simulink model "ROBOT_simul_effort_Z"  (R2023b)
settings: Solver=VariableStepAuto  StartTime=0.0  StopTime=5  RelTol=1e-3
undefined symbols (not defined in the file): deg, kg, m, manette1_Defaut_sldprt, manette2_Defaut_sldprt, mm, N, rad, s, STL, X, Y, Z
libraries: sm_lib x463, fl_lib x45, nesl_utility x27, simulink x2
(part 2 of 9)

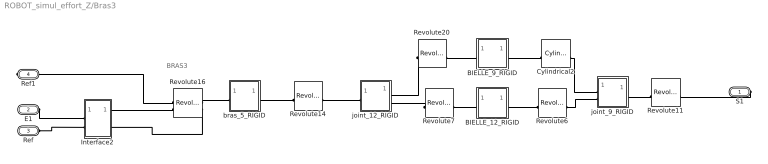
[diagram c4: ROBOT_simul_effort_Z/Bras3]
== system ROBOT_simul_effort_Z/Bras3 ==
  note: BRAS3
  BIELLE_12_RIGID : Subsystem
  BIELLE_9_RIGID : Subsystem
  Cylindrical2 : sm_lib/Joints/Cylindrical Joint  JointMode=Normal  SenseConstraintForce=off  SenseConstraintForceX=off  SenseConstraintForceY=off  SenseConstraintForceZ=off  SenseConstraintTorque=off  SenseConstraintTorqueX=off  SenseConstraintTorqueY=off  SenseConstraintTorqueZ=off  SenseTotalForce=off  SenseTotalForceX=off  SenseTotalForceY=off  SenseTotalForceZ=off  SenseTotalTorque=off  SenseTotalTorqueX=off  SenseTotalTorqueY=off  SenseTotalTorqueZ=off  CompositeWrenchDir=FollowerOnBase  CompositeWrenchFrame=BaseFrame  PzEquilibriumPosition=0  PzEquilibriumPositionUnits=m  PzSpringStiffness=0  PzSpringStiffnessUnits=N/m  PzDampingCoefficient=0  PzDampingCoefficientUnits=s*N/m  PzTorqueActuationMode=NoTorque  PzMotionActuationMode=ComputedMotion  PzSensePosition=off  PzSenseVelocity=off  PzSenseAcceleration=off  PzSenseTorqueForce=off  PzSenseLowerLimitTorqueForce=off  PzSenseUpperLimitTorqueForce=off  PzLowerLimitSpecify=off  PzLowerLimitBound=-1  PzLowerLimitBoundUnits=m  PzLowerLimitStiffness=1e6  PzLowerLimitStiffnessUnits=N/m  PzLowerLimitDamping=1e3  PzLowerLimitDampingUnits=N/(m/s)  PzLowerLimitTransitionRegionWidth=1e-4  PzLowerLimitTransitionRegionWidthUnits=m  PzUpperLimitSpecify=off  PzUpperLimitBound=1  PzUpperLimitBoundUnits=m  PzUpperLimitStiffness=1e6  PzUpperLimitStiffnessUnits=N/m  PzUpperLimitDamping=1e3  PzUpperLimitDampingUnits=N/(m/s)  PzUpperLimitTransitionRegionWidth=1e-4  PzUpperLimitTransitionRegionWidthUnits=m  PzPositionTargetSpecify=off  PzPositionTargetPriority=High  PzPositionTargetValue=0  PzPositionTargetValueUnits=m  PzVelocityTargetSpecify=off  PzVelocityTargetPriority=High  PzVelocityTargetValue=0  PzVelocityTargetValueUnits=m/s  RzEquilibriumPosition=0  RzEquilibriumPositionUnits=rad  RzSpringStiffness=0  RzSpringStiffnessUnits=m*N/rad  RzDampingCoefficient=0  RzDampingCoefficientUnits=m*s*N/rad  RzTorqueActuationMode=NoTorque  RzMotionActuationMode=ComputedMotion  RzSensePosition=off  RzSenseVelocity=off  RzSenseAcceleration=off  RzSenseTorqueForce=off  RzSenseLowerLimitTorqueForce=off  RzSenseUpperLimitTorqueForce=off  RzLowerLimitSpecify=off  RzLowerLimitBound=-90  RzLowerLimitBoundUnits=deg  RzLowerLimitStiffness=1e4  RzLowerLimitStiffnessUnits=N*m/deg  RzLowerLimitDamping=10  RzLowerLimitDampingUnits=N*m/(deg/s)  RzLowerLimitTransitionRegionWidth=0.1  RzLowerLimitTransitionRegionWidthUnits=deg  RzUpperLimitSpecify=off  RzUpperLimitBound=90  RzUpperLimitBoundUnits=deg  RzUpperLimitStiffness=1e4  RzUpperLimitStiffnessUnits=N*m/deg  RzUpperLimitDamping=10  RzUpperLimitDampingUnits=N*m/(deg/s)  RzUpperLimitTransitionRegionWidth=0.1  RzUpperLimitTransitionRegionWidthUnits=deg  RzPositionTargetSpecify=off  RzPositionTargetPriority=High  RzPositionTargetValue=0  RzPositionTargetValueUnits=deg  RzVelocityTargetSpecify=off  RzVelocityTargetPriority=High  RzVelocityTargetValue=0  RzVelocityTargetValueUnits=deg/s
  Interface2 : Subsystem
  Revolute11 : sm_lib/Joints/Revolute Joint  JointMode=Normal  SenseConstraintForce=off  SenseConstraintForceX=off  SenseConstraintForceY=off  SenseConstraintForceZ=off  SenseConstraintTorque=off  SenseConstraintTorqueX=off  SenseConstraintTorqueY=off  SenseConstraintTorqueZ=off  SenseTotalForce=off  SenseTotalForceX=off  SenseTotalForceY=off  SenseTotalForceZ=off  SenseTotalTorque=off  SenseTotalTorqueX=off  SenseTotalTorqueY=off  SenseTotalTorqueZ=off  CompositeWrenchDir=FollowerOnBase  CompositeWrenchFrame=BaseFrame  EquilibriumPosition=0  EquilibriumPositionUnits=rad  SpringStiffness=0  SpringStiffnessUnits=m*N/rad  DampingCoefficient=0  DampingCoefficientUnits=m*s*N/rad  TorqueActuationMode=NoTorque  MotionActuationMode=ComputedMotion  SensePosition=off  SenseVelocity=off  SenseAcceleration=off  SenseTorqueForce=off  SenseLowerLimitTorqueForce=off  SenseUpperLimitTorqueForce=off  LowerLimitSpecify=off  LowerLimitBound=-90  LowerLimitBoundUnits=deg  LowerLimitStiffness=1e4  LowerLimitStiffnessUnits=N*m/deg  LowerLimitDamping=10  LowerLimitDampingUnits=N*m/(deg/s)  LowerLimitTransitionRegionWidth=0.1  LowerLimitTransitionRegionWidthUnits=deg  UpperLimitSpecify=off  UpperLimitBound=90  UpperLimitBoundUnits=deg  UpperLimitStiffness=1e4  UpperLimitStiffnessUnits=N*m/deg  UpperLimitDamping=10  UpperLimitDampingUnits=N*m/(deg/s)  UpperLimitTransitionRegionWidth=0.1  UpperLimitTransitionRegionWidthUnits=deg  PositionTargetSpecify=on  PositionTargetPriority=Low  PositionTargetValue=36.757042846011267  PositionTargetValueUnits=deg  VelocityTargetSpecify=off  VelocityTargetPriority=High  VelocityTargetValue=0  VelocityTargetValueUnits=deg/s
  Revolute14 : sm_lib/Joints/Revolute Joint  JointMode=Normal  SenseConstraintForce=off  SenseConstraintForceX=off  SenseConstraintForceY=off  SenseConstraintForceZ=off  SenseConstraintTorque=off  SenseConstraintTorqueX=off  SenseConstraintTorqueY=off  SenseConstraintTorqueZ=off  SenseTotalForce=off  SenseTotalForceX=off  SenseTotalForceY=off  SenseTotalForceZ=off  SenseTotalTorque=off  SenseTotalTorqueX=off  SenseTotalTorqueY=off  SenseTotalTorqueZ=off  CompositeWrenchDir=FollowerOnBase  CompositeWrenchFrame=BaseFrame  EquilibriumPosition=0  EquilibriumPositionUnits=rad  SpringStiffness=0  SpringStiffnessUnits=m*N/rad  DampingCoefficient=0  DampingCoefficientUnits=m*s*N/rad  TorqueActuationMode=NoTorque  MotionActuationMode=ComputedMotion  SensePosition=off  SenseVelocity=off  SenseAcceleration=off  SenseTorqueForce=off  SenseLowerLimitTorqueForce=off  SenseUpperLimitTorqueForce=off  LowerLimitSpecify=off  LowerLimitBound=-90  LowerLimitBoundUnits=deg  LowerLimitStiffness=1e4  LowerLimitStiffnessUnits=N*m/deg  LowerLimitDamping=10  LowerLimitDampingUnits=N*m/(deg/s)  LowerLimitTransitionRegionWidth=0.1  LowerLimitTransitionRegionWidthUnits=deg  UpperLimitSpecify=off  UpperLimitBound=90  UpperLimitBoundUnits=deg  UpperLimitStiffness=1e4  UpperLimitStiffnessUnits=N*m/deg  UpperLimitDamping=10  UpperLimitDampingUnits=N*m/(deg/s)  UpperLimitTransitionRegionWidth=0.1  UpperLimitTransitionRegionWidthUnits=deg  PositionTargetSpecify=on  PositionTargetPriority=Low  PositionTargetValue=114.86123956506862  PositionTargetValueUnits=deg  VelocityTargetSpecify=off  VelocityTargetPriority=High  VelocityTargetValue=0  VelocityTargetValueUnits=deg/s
  Revolute16 : sm_lib/Joints/Revolute Joint  JointMode=Normal  SenseConstraintForce=off  SenseConstraintForceX=off  SenseConstraintForceY=off  SenseConstraintForceZ=off  SenseConstraintTorque=off  SenseConstraintTorqueX=off  SenseConstraintTorqueY=off  SenseConstraintTorqueZ=off  SenseTotalForce=off  SenseTotalForceX=off  SenseTotalForceY=off  SenseTotalForceZ=off  SenseTotalTorque=off  SenseTotalTorqueX=off  SenseTotalTorqueY=off  SenseTotalTorqueZ=off  CompositeWrenchDir=FollowerOnBase  CompositeWrenchFrame=BaseFrame  EquilibriumPosition=0  EquilibriumPositionUnits=rad  SpringStiffness=0  SpringStiffnessUnits=m*N/rad  DampingCoefficient=0  DampingCoefficientUnits=m*s*N/rad  TorqueActuationMode=InputTorque  MotionActuationMode=ComputedMotion  SensePosition=off  SenseVelocity=on  SenseAcceleration=off  SenseTorqueForce=off  SenseLowerLimitTorqueForce=off  SenseUpperLimitTorqueForce=off  LowerLimitSpecify=off  LowerLimitBound=-90  LowerLimitBoundUnits=deg  LowerLimitStiffness=1e4  LowerLimitStiffnessUnits=N*m/deg  LowerLimitDamping=10  LowerLimitDampingUnits=N*m/(deg/s)  LowerLimitTransitionRegionWidth=0.1  LowerLimitTransitionRegionWidthUnits=deg  UpperLimitSpecify=off  UpperLimitBound=90  UpperLimitBoundUnits=deg  UpperLimitStiffness=1e4  UpperLimitStiffnessUnits=N*m/deg  UpperLimitDamping=10  UpperLimitDampingUnits=N*m/(deg/s)  UpperLimitTransitionRegionWidth=0.1  UpperLimitTransitionRegionWidthUnits=deg  PositionTargetSpecify=on  PositionTargetPriority=Low  PositionTargetValue=101.89580328094226  PositionTargetValueUnits=deg  VelocityTargetSpecify=off  VelocityTargetPriority=High  VelocityTargetValue=0  VelocityTargetValueUnits=deg/s
  Revolute20 : sm_lib/Joints/Revolute Joint  JointMode=Normal  SenseConstraintForce=off  SenseConstraintForceX=off  SenseConstraintForceY=off  SenseConstraintForceZ=off  SenseConstraintTorque=off  SenseConstraintTorqueX=off  SenseConstraintTorqueY=off  SenseConstraintTorqueZ=off  SenseTotalForce=off  SenseTotalForceX=off  SenseTotalForceY=off  SenseTotalForceZ=off  SenseTotalTorque=off  SenseTotalTorqueX=off  SenseTotalTorqueY=off  SenseTotalTorqueZ=off  CompositeWrenchDir=FollowerOnBase  CompositeWrenchFrame=BaseFrame  EquilibriumPosition=0  EquilibriumPositionUnits=rad  SpringStiffness=0  SpringStiffnessUnits=m*N/rad  DampingCoefficient=0  DampingCoefficientUnits=m*s*N/rad  TorqueActuationMode=NoTorque  MotionActuationMode=ComputedMotion  SensePosition=off  SenseVelocity=off  SenseAcceleration=off  SenseTorqueForce=off  SenseLowerLimitTorqueForce=off  SenseUpperLimitTorqueForce=off  LowerLimitSpecify=off  LowerLimitBound=-90  LowerLimitBoundUnits=deg  LowerLimitStiffness=1e4  LowerLimitStiffnessUnits=N*m/deg  LowerLimitDamping=10  LowerLimitDampingUnits=N*m/(deg/s)  LowerLimitTransitionRegionWidth=0.1  LowerLimitTransitionRegionWidthUnits=deg  UpperLimitSpecify=off  UpperLimitBound=90  UpperLimitBoundUnits=deg  UpperLimitStiffness=1e4  UpperLimitStiffnessUnits=N*m/deg  UpperLimitDamping=10  UpperLimitDampingUnits=N*m/(deg/s)  UpperLimitTransitionRegionWidth=0.1  UpperLimitTransitionRegionWidthUnits=deg  PositionTargetSpecify=on  PositionTargetPriority=Low  PositionTargetValue=-178.83470303505044  PositionTargetValueUnits=deg  VelocityTargetSpecify=off  VelocityTargetPriority=High  VelocityTargetValue=0  VelocityTargetValueUnits=deg/s
  Revolute6 : sm_lib/Joints/Revolute Joint  JointMode=Normal  SenseConstraintForce=off  SenseConstraintForceX=off  SenseConstraintForceY=off  SenseConstraintForceZ=off  SenseConstraintTorque=off  SenseConstraintTorqueX=off  SenseConstraintTorqueY=off  SenseConstraintTorqueZ=off  SenseTotalForce=off  SenseTotalForceX=off  SenseTotalForceY=off  SenseTotalForceZ=off  SenseTotalTorque=off  SenseTotalTorqueX=off  SenseTotalTorqueY=off  SenseTotalTorqueZ=off  CompositeWrenchDir=FollowerOnBase  CompositeWrenchFrame=BaseFrame  EquilibriumPosition=0  EquilibriumPositionUnits=rad  SpringStiffness=0  SpringStiffnessUnits=m*N/rad  DampingCoefficient=0  DampingCoefficientUnits=m*s*N/rad  TorqueActuationMode=NoTorque  MotionActuationMode=ComputedMotion  SensePosition=off  SenseVelocity=off  SenseAcceleration=off  SenseTorqueForce=off  SenseLowerLimitTorqueForce=off  SenseUpperLimitTorqueForce=off  LowerLimitSpecify=off  LowerLimitBound=-90  LowerLimitBoundUnits=deg  LowerLimitStiffness=1e4  LowerLimitStiffnessUnits=N*m/deg  LowerLimitDamping=10  LowerLimitDampingUnits=N*m/(deg/s)  LowerLimitTransitionRegionWidth=0.1  LowerLimitTransitionRegionWidthUnits=deg  UpperLimitSpecify=off  UpperLimitBound=90  UpperLimitBoundUnits=deg  UpperLimitStiffness=1e4  UpperLimitStiffnessUnits=N*m/deg  UpperLimitDamping=10  UpperLimitDampingUnits=N*m/(deg/s)  UpperLimitTransitionRegionWidth=0.1  UpperLimitTransitionRegionWidthUnits=deg  PositionTargetSpecify=on  PositionTargetPriority=Low  PositionTargetValue=-178.83470303504936  PositionTargetValueUnits=deg  VelocityTargetSpecify=off  VelocityTargetPriority=High  VelocityTargetValue=0  VelocityTargetValueUnits=deg/s
  Revolute7 : sm_lib/Joints/Revolute Joint  JointMode=Normal  SenseConstraintForce=off  SenseConstraintForceX=off  SenseConstraintForceY=off  SenseConstraintForceZ=off  SenseConstraintTorque=off  SenseConstraintTorqueX=off  SenseConstraintTorqueY=off  SenseConstraintTorqueZ=off  SenseTotalForce=off  SenseTotalForceX=off  SenseTotalForceY=off  SenseTotalForceZ=off  SenseTotalTorque=off  SenseTotalTorqueX=off  SenseTotalTorqueY=off  SenseTotalTorqueZ=off  CompositeWrenchDir=FollowerOnBase  CompositeWrenchFrame=BaseFrame  EquilibriumPosition=0  EquilibriumPositionUnits=rad  SpringStiffness=0  SpringStiffnessUnits=m*N/rad  DampingCoefficient=0  DampingCoefficientUnits=m*s*N/rad  TorqueActuationMode=NoTorque  MotionActuationMode=ComputedMotion  SensePosition=off  SenseVelocity=off  SenseAcceleration=off  SenseTorqueForce=off  SenseLowerLimitTorqueForce=off  SenseUpperLimitTorqueForce=off  LowerLimitSpecify=off  LowerLimitBound=-90  LowerLimitBoundUnits=deg  LowerLimitStiffness=1e4  LowerLimitStiffnessUnits=N*m/deg  LowerLimitDamping=10  LowerLimitDampingUnits=N*m/(deg/s)  LowerLimitTransitionRegionWidth=0.1  LowerLimitTransitionRegionWidthUnits=deg  UpperLimitSpecify=off  UpperLimitBound=90  UpperLimitBoundUnits=deg  UpperLimitStiffness=1e4  UpperLimitStiffnessUnits=N*m/deg  UpperLimitDamping=10  UpperLimitDampingUnits=N*m/(deg/s)  UpperLimitTransitionRegionWidth=0.1  UpperLimitTransitionRegionWidthUnits=deg  PositionTargetSpecify=on  PositionTargetPriority=Low  PositionTargetValue=1.1652969649496245  PositionTargetValueUnits=deg  VelocityTargetSpecify=off  VelocityTargetPriority=High  VelocityTargetValue=0  VelocityTargetValueUnits=deg/s
  bras_5_RIGID : Subsystem
  joint_12_RIGID : Subsystem
  joint_9_RIGID : Subsystem
  S1 : PMIOPort  Side=Right
  E1 : PMIOPort  Port=2  Side=Left
  Ref : PMIOPort  Port=3  Side=Left
  Ref1 : PMIOPort  Port=4  Side=Right
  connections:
  Interface2/RConn2 -- Revolute16/RConn2
  Interface2/RConn1 -- Revolute16/LConn2
  E1/RConn1 -- Interface2/LConn1
  Ref/RConn1 -- Interface2/LConn2
  Revolute11/RConn1 -- joint_9_RIGID/RConn1
  Revolute7/RConn1 -- joint_12_RIGID/RConn2
  Revolute14/RConn1 -- joint_12_RIGID/LConn1
  S1/RConn1 -- Revolute11/LConn1
  Revolute14/LConn1 -- bras_5_RIGID/RConn1
  Revolute16/LConn1 -- Ref1/RConn1
  Revolute16/RConn1 -- bras_5_RIGID/LConn1
  Revolute6/LConn1 -- BIELLE_12_RIGID/RConn1
  BIELLE_12_RIGID/LConn1 -- Revolute7/LConn1
  Revolute6/RConn1 -- joint_9_RIGID/LConn2
  Revolute20/RConn1 -- joint_12_RIGID/RConn1
  BIELLE_9_RIGID/LConn1 -- Revolute20/LConn1
  BIELLE_9_RIGID/RConn1 -- Cylindrical2/LConn1
  Cylindrical2/RConn1 -- joint_9_RIGID/LConn1

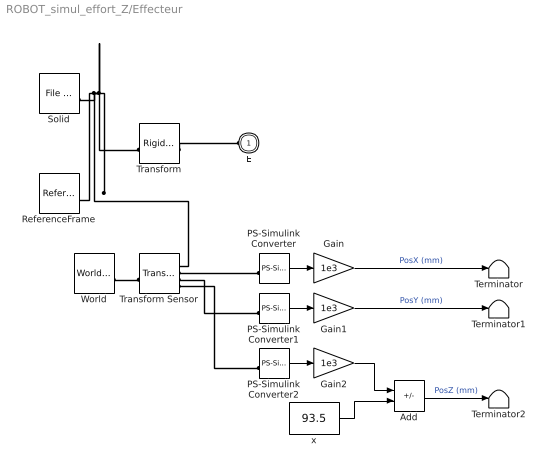
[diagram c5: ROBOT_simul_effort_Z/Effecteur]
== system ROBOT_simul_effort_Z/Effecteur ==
  Add : Sum  Inputs=+-
  Gain : Gain  Gain=1e3
  Gain1 : Gain  Gain=1e3
  Gain2 : Gain  Gain=1e3
  PS-Simulink Converter : nesl_utility/PS-Simulink Converter  PhysicalDomain=network_engine_domain  SubClassName=ps_output  LeftPortType=input  RightPortType=output  PseudoPeriodic=off  Frequencies=[]  VectorFormat=1-D array  Unit=1  AffineConversion=off
  PS-Simulink Converter1 : nesl_utility/PS-Simulink Converter  PhysicalDomain=network_engine_domain  SubClassName=ps_output  LeftPortType=input  RightPortType=output  PseudoPeriodic=off  Frequencies=[]  VectorFormat=1-D array  Unit=1  AffineConversion=off
  PS-Simulink Converter2 : nesl_utility/PS-Simulink Converter  PhysicalDomain=network_engine_domain  SubClassName=ps_output  LeftPortType=input  RightPortType=output  PseudoPeriodic=off  Frequencies=[]  VectorFormat=1-D array  Unit=1  AffineConversion=off
  ReferenceFrame : sm_lib/Frames and Transforms/Reference Frame
  Solid : sm_lib/Body Elements/File Solid  ExtGeomFileName=\STL\manette2_Defaut_sldprt.STL  UnitType=Custom  ExtGeomFileUnits=mm  StepReaderType=HEX  ExportConvexHullGeometry=off  InertiaType=Custom  Mass=0.053  MassUnits=kg  CenterOfMass=[0 0 35.7]  CenterOfMassUnits=mm  MomentsOfInertia=[11.53195593564609 11.464562757624146 11.477456236480506]  MomentsOfInertiaUnits=kg*mm^2  ProductsOfInertia=[-0.014032469477280249 0.0038968914795150661 0.025527028661124163]  ProductsOfInertiaUnits=kg*mm^2  BasedOnType=Density  Density=1000  DensityUnits=kg/(m^3)  DoExposeReferenceFrame=on  SerializedFrames=<Frames/>  GraphicType=FromGeometry  MarkerShape=Sphere  MarkerSize=10  MarkerSizeUnits=m  GraphicVisPropType=SimpleVisualProperties  GraphicDiffuseColor=[1 1 1]  GraphicSpecularColor=[0.5 0.5 0.5 1.0]  GraphicAmbientColor=[0.15 0.15 0.15 1.0]  GraphicEmissiveColor=[0.0 0.0 0.0 1.0]  GraphicShininess=75  GraphicOpacity=1
  Terminator : Terminator
  Terminator1 : Terminator
  Terminator2 : Terminator
  Transform : sm_lib/Frames and Transforms/Rigid Transform  TranslationMethod=Cartesian  TranslationStandardOffset=0  TranslationStandardOffsetUnits=mm  TranslationStandardAxis=+Z  TranslationCartesianOffset=[-0.52204305767083048 1.5422448888264837 -2.2456176397956377e-14]  TranslationCartesianOffsetUnits=mm  TranslationROffset=0  TranslationROffsetUnits=m  TranslationZOffset=0  TranslationZOffsetUnits=m  TranslationThetaOffset=0  TranslationThetaOffsetUnits=deg  RotationMethod=ArbitraryAxis  RotationAngleUnits=rad  RotationStandardAxis=+Z  RotationAngle=2.2920311904365782  RotationArbitraryAxis=[0.63063758405056181 -0.45231899713116352 0.63063758405056158]  FollAlignAxisA=+X  BaseAlignAxisA=+Y  FollAlignAxisB=+Y  BaseAlignAxisB=+Z  RotationSequenceAxes=FollowerAxes  RotationSequence=XYX  RotationSequenceAngles=[0 0 0]  RotationSequenceAnglesUnits=deg  RotationMatrix=[1 0 0; 0 1 0; 0 0 1]  Quaternion=[1 0 0 0]
  Transform Sensor : sm_lib/Frames and Transforms/Transform Sensor  MeasurementFrame=World  RotationSequence=XYX  SenseAngle=off  SenseAxis=off  SenseQ=off  SenseR=off  SenseRotationSequence=off  SenseOmegaX=off  SenseOmegaY=off  SenseOmegaZ=off  SenseOmega=off  SenseQDot=off  SenseRDot=off  SenseRotationSequenceDot=off  SenseAlphaX=off  SenseAlphaY=off  SenseAlphaZ=off  SenseAlpha=off  SenseQDDot=off  SenseRDDot=off  SenseX=on  SenseY=on  SenseZ=on  SenseXYZ=off  SenseRad=off  SenseAzim=off  SenseDist=off  SenseInc=off  SenseXDot=off  SenseYDot=off  SenseZDot=off  SenseXYZDot=off  SenseRadDot=off  SenseAzimDot=off  SenseDistDot=off  SenseIncDot=off  SenseXDDot=off  SenseYDDot=off  SenseZDDot=off  SenseXYZDDot=off  SenseRadDDot=off  SenseAzimDDot=off  SenseDistDDot=off  SenseIncDDot=off
  World : sm_lib/Frames and Transforms/World Frame
  x : Constant  Value=93.5
  E : PMIOPort  Side=Left
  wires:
  Gain1/1 -> Terminator1/1  "PosY (mm)"
  PS-Simulink Converter2/1 -> Gain2/1
  x/1 -> Add/2
  Add/1 -> Terminator2/1  "PosZ (mm)"
  PS-Simulink Converter1/1 -> Gain1/1
  Gain2/1 -> Add/1
  PS-Simulink Converter/1 -> Gain/1
  Gain/1 -> Terminator/1  "PosX (mm)"
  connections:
  Solid/RConn1 -- ReferenceFrame/RConn1 -- Transform Sensor/RConn1 -- Transform/LConn1
  Transform/RConn1 -- E/RConn1
  Transform Sensor/RConn3 -- PS-Simulink Converter1/LConn1
  World/RConn1 -- Transform Sensor/LConn1
  PS-Simulink Converter2/LConn1 -- Transform Sensor/RConn4
  Transform Sensor/RConn2 -- PS-Simulink Converter/LConn1

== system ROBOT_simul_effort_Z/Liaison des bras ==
  EFFECTEUR_1_RIGID : Subsystem
  manette_1_RIGID : Subsystem
  E1 : PMIOPort  Side=Left
  E2 : PMIOPort  Port=2  Side=Left
  S1 : PMIOPort  Port=3  Side=Right
  E3 : PMIOPort  Port=4  Side=Left
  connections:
  EFFECTEUR_1_RIGID/RConn1 -- manette_1_RIGID/LConn1
  S1/RConn1 -- manette_1_RIGID/RConn1
  EFFECTEUR_1_RIGID/LConn1 -- E2/RConn1
  EFFECTEUR_1_RIGID/LConn3 -- E1/RConn1
  EFFECTEUR_1_RIGID/LConn2 -- E3/RConn1

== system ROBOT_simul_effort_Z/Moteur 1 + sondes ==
  In1 : Inport
  Moteur courant continu1 : Subsystem
  Reference electrique : fl_lib/Electrical/Electrical Elements/Electrical Reference
  Simulink-PS Converter1 : nesl_utility/Simulink-PS Converter  PhysicalDomain=network_engine_domain  SubClassName=ps_input  LeftPortType=input  RightPortType=output  PseudoPeriodic=off  Frequencies=[]  NoiseDistribution=none  NoiseParameters=[]  Unit=V  AffineConversion=off  FilteringAndDerivatives=zero  SimscapeFilterOrder=2  InputFilterTimeConstant=1e-4  UdotUserProvided=1
  Sondes electriques1 : Subsystem
  Source de tension controlée1 : fl_lib/Electrical/Electrical Sources/Controlled Voltage Source
  Conn1 : PMIOPort  Side=Right
  Conn2 : PMIOPort  Port=2  Side=Right
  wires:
  In1/1 -> Simulink-PS Converter1/1
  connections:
  Conn2/RConn1 -- Moteur courant continu1/RConn2
  Conn1/RConn1 -- Moteur courant continu1/RConn1
  Source de tension controlée1/LConn1 -- Sondes electriques1/LConn1
  Simulink-PS Converter1/RConn1 -- Source de tension controlée1/RConn1
  Sondes electriques1/RConn2 -- Source de tension controlée1/RConn2 -- Reference electrique/LConn1 -- Moteur courant continu1/LConn2
  Sondes electriques1/RConn1 -- Moteur courant continu1/LConn1

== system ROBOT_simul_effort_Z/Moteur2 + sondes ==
  In1 : Inport
  Moteur courant continu2 : Subsystem
  Reference electrique : fl_lib/Electrical/Electrical Elements/Electrical Reference
  Simulink-PS Converter1 : nesl_utility/Simulink-PS Converter  PhysicalDomain=network_engine_domain  SubClassName=ps_input  LeftPortType=input  RightPortType=output  PseudoPeriodic=off  Frequencies=[]  NoiseDistribution=none  NoiseParameters=[]  Unit=V  AffineConversion=off  FilteringAndDerivatives=zero  SimscapeFilterOrder=2  InputFilterTimeConstant=1e-4  UdotUserProvided=1
  Sondes electriques : Subsystem
  Source de tension controlée : fl_lib/Electrical/Electrical Sources/Controlled Voltage Source
  Conn1 : PMIOPort  Side=Right
  Conn2 : PMIOPort  Port=2  Side=Right
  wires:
  In1/1 -> Simulink-PS Converter1/1
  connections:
  Sondes electriques/RConn1 -- Moteur courant continu2/LConn1
  Source de tension controlée/RConn2 -- Reference electrique/LConn1 -- Sondes electriques/RConn2 -- Moteur courant continu2/LConn2
  Simulink-PS Converter1/RConn1 -- Source de tension controlée/RConn1
  Source de tension controlée/LConn1 -- Sondes electriques/LConn1
  Conn1/RConn1 -- Moteur courant continu2/RConn1
  Conn2/RConn1 -- Moteur courant continu2/RConn2

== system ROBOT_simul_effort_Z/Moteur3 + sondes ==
  In1 : Inport
  Moteur courant continu3 : Subsystem
  Reference electrique : fl_lib/Electrical/Electrical Elements/Electrical Reference
  Simulink-PS Converter1 : nesl_utility/Simulink-PS Converter  PhysicalDomain=network_engine_domain  SubClassName=ps_input  LeftPortType=input  RightPortType=output  PseudoPeriodic=off  Frequencies=[]  NoiseDistribution=none  NoiseParameters=[]  Unit=V  AffineConversion=off  FilteringAndDerivatives=zero  SimscapeFilterOrder=2  InputFilterTimeConstant=1e-4  UdotUserProvided=1
  Sondes electriques3 : Subsystem
  Source de tension controlée3 : fl_lib/Electrical/Electrical Sources/Controlled Voltage Source
  Conn1 : PMIOPort  Side=Right
  Conn2 : PMIOPort  Port=2  Side=Right
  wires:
  In1/1 -> Simulink-PS Converter1/1
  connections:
  Sondes electriques3/RConn1 -- Moteur courant continu3/LConn1
  Moteur courant continu3/LConn2 -- Reference electrique/LConn1 -- Source de tension controlée3/RConn2 -- Sondes electriques3/RConn2
  Simulink-PS Converter1/RConn1 -- Source de tension controlée3/RConn1
  Source de tension controlée3/LConn1 -- Sondes electriques3/LConn1
  Conn1/RConn1 -- Moteur courant continu3/RConn1
  Conn2/RConn1 -- Moteur courant continu3/RConn2

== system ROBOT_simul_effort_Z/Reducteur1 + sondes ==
  Conv en tr/s : Gain  Gain=-60/(2*pi)
  Conv w : nesl_utility/PS-Simulink Converter  PhysicalDomain=network_engine_domain  SubClassName=ps_output  LeftPortType=input  RightPortType=output  PseudoPeriodic=off  Frequencies=[]  VectorFormat=1-D array  Unit=1  AffineConversion=off
  Conv w1 : nesl_utility/PS-Simulink Converter  PhysicalDomain=network_engine_domain  SubClassName=ps_output  LeftPortType=input  RightPortType=output  PseudoPeriodic=off  Frequencies=[]  VectorFormat=1-D array  Unit=1  AffineConversion=off
  Invers signe : Gain  Gain=-1
  Reference mecanique : fl_lib/Mechanical/Rotational Elements/Mechanical Rotational Reference
  Rotational Hard Stop : fl_lib/Mechanical/Rotational Elements/Rotational Hard Stop  Commented=on  upper_bnd=0 rad  lower_bnd=-1.95 rad  model=simscape.enum.hardstop.fulldamped  stiff_up=1e+4 N*m/rad  stiff_low=1e+4 N*m/rad  D_up=100 N*m/(rad/s)  D_low=100 N*m/(rad/s)  transition=0.001 rad  coeff_rest=0.7  w_tol=0.1 rad/s  trq_tol=0.001 N*m  w_specify=off  w_priority=None  w=0 rad/s  w_nominal_specify=off  w_nominal_unit=rad/s  w_nominal_value=1  t_specify=off  t_priority=None  t=0 N*m  t_nominal_specify=off  t_nominal_unit=N*m  t_nominal_value=1  phi_specify=on  phi_priority=High  phi=0 rad  phi_nominal_specify=off  phi_nominal_unit=rad  phi_nominal_value=1  M_specify=off  M_priority=None  M=0
  Réducteur de vitesse : fl_lib/Mechanical/Mechanisms/Gear Box  ratio=-7.627  t_in_specify=off  t_in_priority=None  t_in=0 N*m  t_in_nominal_specify=off  t_in_nominal_unit=N*m  t_in_nominal_value=1  t_out_specify=off  t_out_priority=None  t_out=0 N*m  t_out_nominal_specify=off  t_out_nominal_unit=N*m  t_out_nominal_value=1
  Sonde omega /theta1 : fl_lib/Mechanical/Mechanical Sensors/Ideal Rotational Motion Sensor  reference=foundation.enum.MeasurementReference.difference  acceleration_port=false  velocity_port=true  position_port=true  wrap_angle=false  offset=0 rad
  Terminator : Terminator
  Terminator1 : Terminator
  E1 : PMIOPort  Side=Left
  Ref : PMIOPort  Port=2  Side=Left
  S1 : PMIOPort  Port=3  Side=Right
  Ref1 : PMIOPort  Port=4  Side=Right
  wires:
  Conv w1/1 -> Invers signe/1  "Angle_mot1 (rad)"
  Invers signe/1 -> Terminator1/1  "Angle_mot1 (rad)"
  Conv w/1 -> Conv en tr/s/1
  Conv en tr/s/1 -> Terminator/1  "Nmoteur1 (tr/min)"
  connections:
  Sonde omega /theta1/LConn1 -- E1/RConn1 -- Réducteur de vitesse/LConn1
  Reference mecanique/LConn1 -- Ref/RConn1 -- Ref1/RConn1 -- Rotational Hard Stop/RConn1 -- Sonde omega /theta1/RConn1
  Conv w/LConn1 -- Sonde omega /theta1/RConn2
  Conv w1/LConn1 -- Sonde omega /theta1/RConn3
  Réducteur de vitesse/RConn1 -- Rotational Hard Stop/LConn1 -- S1/RConn1

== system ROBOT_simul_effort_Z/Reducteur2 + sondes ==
  Conv en tr/s : Gain  Gain=60/(2*pi)
  Conv en ° : Gain  Gain=180/pi
  Conv w : nesl_utility/PS-Simulink Converter  PhysicalDomain=network_engine_domain  SubClassName=ps_output  LeftPortType=input  RightPortType=output  PseudoPeriodic=off  Frequencies=[]  VectorFormat=1-D array  Unit=1  AffineConversion=off
  Conv w1 : nesl_utility/PS-Simulink Converter  PhysicalDomain=network_engine_domain  SubClassName=ps_output  LeftPortType=input  RightPortType=output  PseudoPeriodic=off  Frequencies=[]  VectorFormat=1-D array  Unit=1  AffineConversion=off
  Reference mecanique : fl_lib/Mechanical/Rotational Elements/Mechanical Rotational Reference
  Rotational Hard Stop : fl_lib/Mechanical/Rotational Elements/Rotational Hard Stop  Commented=on  upper_bnd=1.95 rad  lower_bnd=0 rad  model=simscape.enum.hardstop.fulldamped  stiff_up=1e+4 N*m/rad  stiff_low=1e+4 N*m/rad  D_up=100 N*m/(rad/s)  D_low=100 N*m/(rad/s)  transition=0.001 rad  coeff_rest=0.7  w_tol=0.1 rad/s  trq_tol=0.001 N*m  w_specify=off  w_priority=None  w=0 rad/s  w_nominal_specify=off  w_nominal_unit=rad/s  w_nominal_value=1  t_specify=off  t_priority=None  t=0 N*m  t_nominal_specify=off  t_nominal_unit=N*m  t_nominal_value=1  phi_specify=on  phi_priority=High  phi=0 rad  phi_nominal_specify=off  phi_nominal_unit=rad  phi_nominal_value=1  M_specify=off  M_priority=None  M=0
  Réducteur de vitesse2 : fl_lib/Mechanical/Mechanisms/Gear Box  ratio=7.627  t_in_specify=off  t_in_priority=None  t_in=0 N*m  t_in_nominal_specify=off  t_in_nominal_unit=N*m  t_in_nominal_value=1  t_out_specify=off  t_out_priority=None  t_out=0 N*m  t_out_nominal_specify=off  t_out_nominal_unit=N*m  t_out_nominal_value=1
  Sonde omega /theta2 : fl_lib/Mechanical/Mechanical Sensors/Ideal Rotational Motion Sensor  reference=foundation.enum.MeasurementReference.difference  acceleration_port=false  velocity_port=true  position_port=true  wrap_angle=false  offset=0 rad
  Terminator : Terminator
  Terminator1 : Terminator
  E1 : PMIOPort  Side=Left
  Ref : PMIOPort  Port=2  Side=Left
  S1 : PMIOPort  Port=3  Side=Right
  Ref1 : PMIOPort  Port=4  Side=Right
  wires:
  Conv w1/1 -> Conv en °/1  "Angle_mot2 (rad)"
  Conv en °/1 -> Terminator1/1  "Angle_mot2 (°)"
  Conv w/1 -> Conv en tr/s/1
  Conv en tr/s/1 -> Terminator/1  "Nmoteur2 (tr/min)"
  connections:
  Sonde omega /theta2/LConn1 -- E1/RConn1 -- Réducteur de vitesse2/LConn1
  Ref1/RConn1 -- Sonde omega /theta2/RConn1 -- Reference mecanique/LConn1 -- Ref/RConn1 -- Rotational Hard Stop/RConn1
  Conv w1/LConn1 -- Sonde omega /theta2/RConn3
  Conv w/LConn1 -- Sonde omega /theta2/RConn2
  Réducteur de vitesse2/RConn1 -- Rotational Hard Stop/LConn1 -- S1/RConn1

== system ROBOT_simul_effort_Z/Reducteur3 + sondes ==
  Conv en tr/s : Gain  Gain=60/(2*pi)
  Conv en ° : Gain  Gain=180/pi
  Conv w : nesl_utility/PS-Simulink Converter  PhysicalDomain=network_engine_domain  SubClassName=ps_output  LeftPortType=input  RightPortType=output  PseudoPeriodic=off  Frequencies=[]  VectorFormat=1-D array  Unit=1  AffineConversion=off
  Conv w1 : nesl_utility/PS-Simulink Converter  PhysicalDomain=network_engine_domain  SubClassName=ps_output  LeftPortType=input  RightPortType=output  PseudoPeriodic=off  Frequencies=[]  VectorFormat=1-D array  Unit=1  AffineConversion=off
  Reference mecanique : fl_lib/Mechanical/Rotational Elements/Mechanical Rotational Reference
  Rotational Hard Stop : fl_lib/Mechanical/Rotational Elements/Rotational Hard Stop  Commented=on  upper_bnd=1.95 rad  lower_bnd=0 rad  model=simscape.enum.hardstop.fulldamped  stiff_up=1e+4 N*m/rad  stiff_low=1e+4 N*m/rad  D_up=100 N*m/(rad/s)  D_low=100 N*m/(rad/s)  transition=0.001 rad  coeff_rest=0.7  w_tol=0.1 rad/s  trq_tol=0.001 N*m  w_specify=off  w_priority=None  w=0 rad/s  w_nominal_specify=off  w_nominal_unit=rad/s  w_nominal_value=1  t_specify=off  t_priority=None  t=0 N*m  t_nominal_specify=off  t_nominal_unit=N*m  t_nominal_value=1  phi_specify=on  phi_priority=High  phi=0 rad  phi_nominal_specify=off  phi_nominal_unit=rad  phi_nominal_value=1  M_specify=off  M_priority=None  M=0
  Réducteur de vitesse3 : fl_lib/Mechanical/Mechanisms/Gear Box  ratio=7.627  t_in_specify=off  t_in_priority=None  t_in=0 N*m  t_in_nominal_specify=off  t_in_nominal_unit=N*m  t_in_nominal_value=1  t_out_specify=off  t_out_priority=None  t_out=0 N*m  t_out_nominal_specify=off  t_out_nominal_unit=N*m  t_out_nominal_value=1
  Sonde omega /theta2 : fl_lib/Mechanical/Mechanical Sensors/Ideal Rotational Motion Sensor  reference=foundation.enum.MeasurementReference.difference  acceleration_port=false  velocity_port=true  position_port=true  wrap_angle=false  offset=0 rad
  Terminator : Terminator
  Terminator1 : Terminator
  E1 : PMIOPort  Side=Left
  Ref : PMIOPort  Port=2  Side=Left
  S1 : PMIOPort  Port=3  Side=Right
  Ref1 : PMIOPort  Port=4  Side=Right
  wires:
  Conv w1/1 -> Conv en °/1  "Angle_mot3 (rad)"
  Conv en °/1 -> Terminator1/1  "Angle_mot3 (°)"
  Conv w/1 -> Conv en tr/s/1
  Conv en tr/s/1 -> Terminator/1  "Nmoteur3 (tr/min)"
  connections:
  Sonde omega /theta2/LConn1 -- E1/RConn1 -- Réducteur de vitesse3/LConn1
  Ref/RConn1 -- Reference mecanique/LConn1 -- Rotational Hard Stop/RConn1 -- Ref1/RConn1 -- Sonde omega /theta2/RConn1
  Conv w1/LConn1 -- Sonde omega /theta2/RConn3
  Réducteur de vitesse3/RConn1 -- Rotational Hard Stop/LConn1 -- S1/RConn1
  Conv w/LConn1 -- Sonde omega /theta2/RConn2

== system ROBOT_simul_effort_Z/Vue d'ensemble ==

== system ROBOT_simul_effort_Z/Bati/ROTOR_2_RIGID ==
  CODEUR_1_RIGID : Subsystem
  ROTOR_1_RIGID : Subsystem
  ReferenceFrame : sm_lib/Frames and Transforms/Reference Frame
  Transform : sm_lib/Frames and Transforms/Rigid Transform  TranslationMethod=Cartesian  TranslationStandardOffset=0  TranslationStandardOffsetUnits=mm  TranslationStandardAxis=+Z  TranslationCartesianOffset=[30.900000000000009 0 -2.4868995751603507e-14]  TranslationCartesianOffsetUnits=mm  TranslationROffset=0  TranslationROffsetUnits=m  TranslationZOffset=0  TranslationZOffsetUnits=m  TranslationThetaOffset=0  TranslationThetaOffsetUnits=deg  RotationMethod=ArbitraryAxis  RotationAngleUnits=rad  RotationStandardAxis=+Z  RotationAngle=2.0943951023931953  RotationArbitraryAxis=[0.57735026918962584 0.57735026918962562 0.57735026918962584]  FollAlignAxisA=+X  BaseAlignAxisA=+Y  FollAlignAxisB=+Y  BaseAlignAxisB=+Z  RotationSequenceAxes=FollowerAxes  RotationSequence=XYX  RotationSequenceAngles=[0 0 0]  RotationSequenceAnglesUnits=deg  RotationMatrix=[1 0 0; 0 1 0; 0 0 1]  Quaternion=[1 0 0 0]
  Transform1 : sm_lib/Frames and Transforms/Rigid Transform  TranslationMethod=Cartesian  TranslationStandardOffset=0  TranslationStandardOffsetUnits=mm  TranslationStandardAxis=+Z  TranslationCartesianOffset=[30.899999999999991 0 0]  TranslationCartesianOffsetUnits=mm  TranslationROffset=0  TranslationROffsetUnits=m  TranslationZOffset=0  TranslationZOffsetUnits=m  TranslationThetaOffset=0  TranslationThetaOffsetUnits=deg  RotationMethod=ArbitraryAxis  RotationAngleUnits=rad  RotationStandardAxis=+Z  RotationAngle=1.9381695666920589  RotationArbitraryAxis=[0.51405666735189148 -0.51405666735189148 0.68665237602598705]  FollAlignAxisA=+X  BaseAlignAxisA=+Y  FollAlignAxisB=+Y  BaseAlignAxisB=+Z  RotationSequenceAxes=FollowerAxes  RotationSequence=XYX  RotationSequenceAngles=[0 0 0]  RotationSequenceAnglesUnits=deg  RotationMatrix=[1 0 0; 0 1 0; 0 0 1]  Quaternion=[1 0 0 0]
  Transform2 : sm_lib/Frames and Transforms/Rigid Transform  TranslationMethod=Cartesian  TranslationStandardOffset=0  TranslationStandardOffsetUnits=mm  TranslationStandardAxis=+Z  TranslationCartesianOffset=[-36.399999999999999 0 0]  TranslationCartesianOffsetUnits=mm  TranslationROffset=0  TranslationROffsetUnits=m  TranslationZOffset=0  TranslationZOffsetUnits=m  TranslationThetaOffset=0  TranslationThetaOffsetUnits=deg  RotationMethod=ArbitraryAxis  RotationAngleUnits=rad  RotationStandardAxis=+Z  RotationAngle=1.624664356272121  RotationArbitraryAxis=[-0.22603347840136132 0.22603347840136129 0.94753244444903439]  FollAlignAxisA=+X  BaseAlignAxisA=+Y  FollAlignAxisB=+Y  BaseAlignAxisB=+Z  RotationSequenceAxes=FollowerAxes  RotationSequence=XYX  RotationSequenceAngles=[0 0 0]  RotationSequenceAnglesUnits=deg  RotationMatrix=[1 0 0; 0 1 0; 0 0 1]  Quaternion=[1 0 0 0]
  F : PMIOPort  Side=Left
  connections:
  ReferenceFrame/RConn1 -- Transform/LConn1 -- Transform1/LConn1 -- Transform2/LConn1
  Transform/RConn1 -- F/RConn1
  ROTOR_1_RIGID/LConn1 -- Transform1/RConn1
  CODEUR_1_RIGID/LConn1 -- Transform2/RConn1

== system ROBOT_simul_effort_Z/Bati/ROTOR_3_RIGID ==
  CODEUR_1_RIGID : Subsystem
  ROTOR_1_RIGID : Subsystem
  ReferenceFrame : sm_lib/Frames and Transforms/Reference Frame
  Transform : sm_lib/Frames and Transforms/Rigid Transform  TranslationMethod=Cartesian  TranslationStandardOffset=0  TranslationStandardOffsetUnits=mm  TranslationStandardAxis=+Z  TranslationCartesianOffset=[30.899999999999984 -7.1054273576010019e-15 1.7763568394002505e-15]  TranslationCartesianOffsetUnits=mm  TranslationROffset=0  TranslationROffsetUnits=m  TranslationZOffset=0  TranslationZOffsetUnits=m  TranslationThetaOffset=0  TranslationThetaOffsetUnits=deg  RotationMethod=ArbitraryAxis  RotationAngleUnits=rad  RotationStandardAxis=+Z  RotationAngle=2.0943951023931953  RotationArbitraryAxis=[0.57735026918962562 0.57735026918962584 0.57735026918962595]  FollAlignAxisA=+X  BaseAlignAxisA=+Y  FollAlignAxisB=+Y  BaseAlignAxisB=+Z  RotationSequenceAxes=FollowerAxes  RotationSequence=XYX  RotationSequenceAngles=[0 0 0]  RotationSequenceAnglesUnits=deg  RotationMatrix=[1 0 0; 0 1 0; 0 0 1]  Quaternion=[1 0 0 0]
  Transform1 : sm_lib/Frames and Transforms/Rigid Transform  TranslationMethod=Cartesian  TranslationStandardOffset=0  TranslationStandardOffsetUnits=mm  TranslationStandardAxis=+Z  TranslationCartesianOffset=[30.899999999999999 0 0]  TranslationCartesianOffsetUnits=mm  TranslationROffset=0  TranslationROffsetUnits=m  TranslationZOffset=0  TranslationZOffsetUnits=m  TranslationThetaOffset=0  TranslationThetaOffsetUnits=deg  RotationMethod=ArbitraryAxis  RotationAngleUnits=rad  RotationStandardAxis=+Z  RotationAngle=1.9381695666920589  RotationArbitraryAxis=[0.51405666735189148 -0.51405666735189148 0.68665237602598705]  FollAlignAxisA=+X  BaseAlignAxisA=+Y  FollAlignAxisB=+Y  BaseAlignAxisB=+Z  RotationSequenceAxes=FollowerAxes  RotationSequence=XYX  RotationSequenceAngles=[0 0 0]  RotationSequenceAnglesUnits=deg  RotationMatrix=[1 0 0; 0 1 0; 0 0 1]  Quaternion=[1 0 0 0]
  Transform2 : sm_lib/Frames and Transforms/Rigid Transform  TranslationMethod=Cartesian  TranslationStandardOffset=0  TranslationStandardOffsetUnits=mm  TranslationStandardAxis=+Z  TranslationCartesianOffset=[-36.399999999999999 0 0]  TranslationCartesianOffsetUnits=mm  TranslationROffset=0  TranslationROffsetUnits=m  TranslationZOffset=0  TranslationZOffsetUnits=m  TranslationThetaOffset=0  TranslationThetaOffsetUnits=deg  RotationMethod=ArbitraryAxis  RotationAngleUnits=rad  RotationStandardAxis=+Z  RotationAngle=1.624664356272121  RotationArbitraryAxis=[-0.22603347840136134 0.22603347840136132 0.94753244444903439]  FollAlignAxisA=+X  BaseAlignAxisA=+Y  FollAlignAxisB=+Y  BaseAlignAxisB=+Z  RotationSequenceAxes=FollowerAxes  RotationSequence=XYX  RotationSequenceAngles=[0 0 0]  RotationSequenceAnglesUnits=deg  RotationMatrix=[1 0 0; 0 1 0; 0 0 1]  Quaternion=[1 0 0 0]
  F : PMIOPort  Side=Left
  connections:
  Transform/LConn1 -- ReferenceFrame/RConn1 -- Transform1/LConn1 -- Transform2/LConn1
  Transform/RConn1 -- F/RConn1
  ROTOR_1_RIGID/LConn1 -- Transform1/RConn1
  CODEUR_1_RIGID/LConn1 -- Transform2/RConn1
